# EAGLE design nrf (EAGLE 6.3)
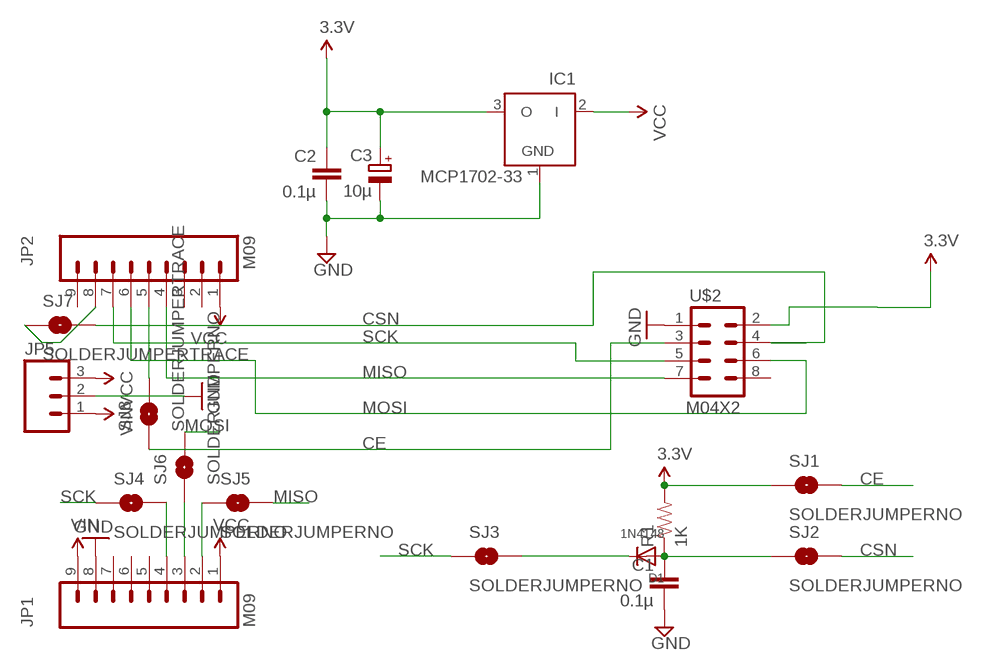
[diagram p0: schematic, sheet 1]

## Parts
C1  0.1µ  CAPPTH  [CAP-PTH-SMALL]
C2  0.1µ  CAPPTH  [CAP-PTH-SMALL]
C3  10µ  CPOL-EUE1.8-4  [E1,8-4]
D1  1N4148  DIODEDO-1N4148  [DO-1N4148]
IC1  MCP1702-33  MCP1702Z  [TO92]
JP1  M09  [1X09]
JP2  M09  [1X09]
JP5  M03PTH  [1X03]
R1  1K  RESISTORAXIAL-0.3  [AXIAL-0.3]
SJ1  SOLDERJUMPERNO  [SJ_2S-NO]
SJ2  SOLDERJUMPERNO  [SJ_2S-NO]
SJ3  SOLDERJUMPERNO  [SJ_2S-NO]
SJ4  SOLDERJUMPERNO  [SJ_2S-NO]
SJ5  SOLDERJUMPERNO  [SJ_2S-NO]
SJ6  SOLDERJUMPERNO  [SJ_2S-NO]
SJ7  SOLDERJUMPERTRACE  [SJ_2S-TRACE]
SJ8  SOLDERJUMPERTRACE  [SJ_2S-TRACE]
U$2  M04X2  [2X4]

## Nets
3.3V: C2.1 C3.+ IC1.3(O) R1.P$2 SJ1.1 U$2.2
CE: SJ1.2 SJ8.1 U$2.3
CSN: SJ2.2 SJ7.2 U$2.4
GND [POWER]: C1.2 C2.2 C3.- IC1.1(GND) JP1.8 JP5.2 U$2.1
MISO: JP2.4 SJ5.2 U$2.7
MOSI: JP2.6 SJ6.2 U$2.6
N$1: C1.1 D1.A R1.P$1 SJ2.1
N$2: JP2.8 SJ7.1
N$3: JP2.5 SJ8.2
N$7: D1.C SJ3.2
N$8: JP1.2 SJ5.1
N$9: JP1.3 SJ6.1
N$10: JP1.4 SJ4.2
SCK: JP2.7 SJ3.1 SJ4.1 U$2.5
VCC [POWER]: IC1.2(I) JP1.1 JP2.1 JP5.3
VIN [POWER]: JP1.9 JP5.1
Unconnected: JP1.5 JP1.6 JP1.7 JP2.2 JP2.3 JP2.9 U$2.8

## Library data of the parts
C1 C2 = SparkFun:CAP: Capacitor
C3 = resistor:CPOL-EU: POLARIZED CAPACITOR, European symbol
D1 = adafruit:DIODE: Diode
IC1 = JeeLabs:MCP1702: 200 mA, Low Power Low Dropout Voltage Regulator
JP1 JP2 = SparkFun:M09: Header 9 Standard 9-pin 0.1" header. Use with straight break away headers (SKU : PRT-00116), right angle break away headers (PRT-00553), swiss pins (PRT-00743), machine pins (PRT-00117), and female headers (PRT-00115).
JP5 = SparkFun:M03: Header 3 Standard 3-pin 0.1" header. Use with straight break away headers (SKU : PRT-00116), right angle break away headers (PRT-00553), swiss pins (PRT-00743), machine pins (PRT-00117), and female headers (PRT-00115). Molex polarized connector foot print use with SKU : PRT-08232 with associated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
R1 = SparkFun-Passives:RESISTOR: Resistor
SJ1-SJ8 = SparkFun-Passives:SOLDERJUMPER: Solder Jumper
U$2 = SparkFun-Connectors:M04X2: .1" header, two rows of four.

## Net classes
0 default: width 0.203 mm
1 POWER: width 0.203 mm

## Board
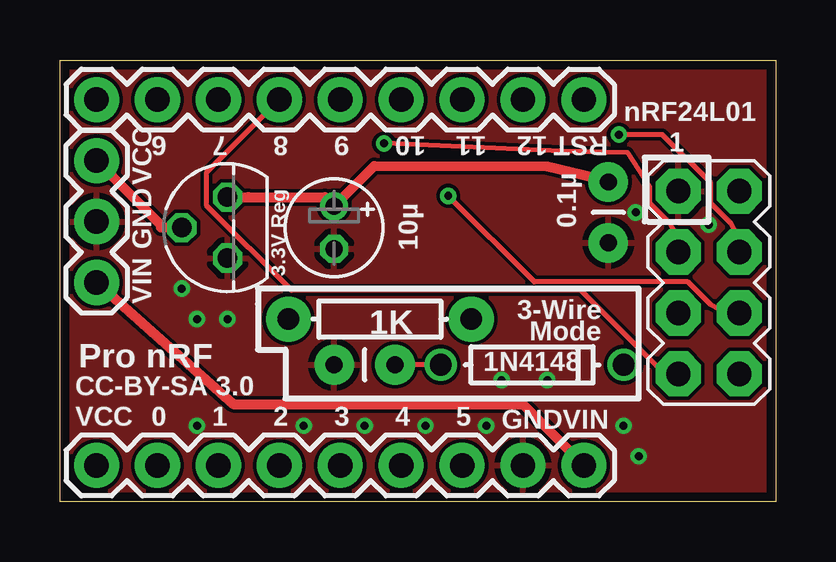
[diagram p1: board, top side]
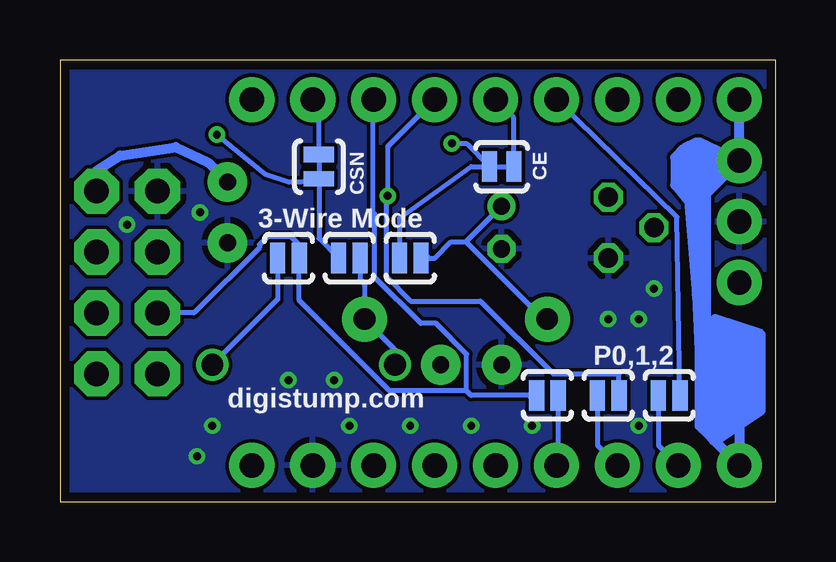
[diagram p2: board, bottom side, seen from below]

Size 29.84 x 18.41 mm. Coordinates in mm from the lower left corner, seen from the top.
Outline: 0,0 0,18.41 29.84,18.41 29.84,0 0,0
Copper layers (1*16): Top 0.0356mm / dielectric 1.5011mm / Bottom 0.0356mm
Design rules "eriks *": minimum track width 8mil, minimum drill 13mil, track to track 6mil, track to pad 6mil, pad to pad 6mil, via to via 6mil, smd to smd 6mil, copper to edge 15mil, drill to drill 6mil, minimum pad ring 7mil, minimum via ring 7mil, stop-mask expansion 4mil, vias tented up to drill 20mil, thermal gap 10mil

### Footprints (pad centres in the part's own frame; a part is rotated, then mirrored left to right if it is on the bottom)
CAP-PTH-SMALL = drill 0.7 pad 1.651: 1 0,0; 2 2.54,0
E1,8-4 = drill 0.711 pad 1.168: + -0.889,0 | drill 0.711 pad 1.168 octagon: - 0.889,0
DO-1N4148 = drill 0.9: A -3.81,0; C 3.81,0
TO92 = drill 0.813 octagon: 1 -1.27,0; 2 0,1.905; 3 1.27,0
1X09 = drill 1.016 pad 1.88: 1 0,0; 2 2.54,0; 3 5.08,0; 4 7.62,0; 5 10.16,0; 6 12.7,0; 7 15.24,0; 8 17.78,0; 9 20.32,0
1X03 = drill 1.016 pad 1.88: 1 0,0; 2 2.54,0; 3 5.08,0
AXIAL-0.3 = drill 0.9 pad 1.88: P$1 -3.81,0; P$2 3.81,0
SJ_2S-NO = smd 0.635 x 1.27: 1 -0.45,0; 2 0.45,0
SJ_2S-TRACE = smd 0.635 x 1.27: 1 -0.508,0; 2 0.508,0
2X4 = drill 1.016 pad 1.88 octagon: 1 -3.81,-1.27; 2 -3.81,1.27; 3 -1.27,-1.27; 4 -1.27,1.27; 5 1.27,-1.27; 6 1.27,1.27; 7 3.81,-1.27; 8 3.81,1.27

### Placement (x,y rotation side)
C1  13.97,5.71 180 top
C2  22.86,13.34 270 top
C3  11.43,11.43 270 top
D1  19.68,5.71 0 top
IC1  6.99,11.43 90 top
JP1  1.52,1.52 0 top
JP2  1.52,16.76 0 top
JP5  1.52,9.14 90 top
R1  13.34,7.62 180 top
SJ1  15.24,10.16 180 bottom
SJ2  17.78,10.16 180 bottom
SJ3  20.32,10.16 180 bottom
SJ4  9.53,4.45 0 bottom
SJ5  4.45,4.45 0 bottom
SJ6  6.99,4.45 0 bottom
SJ7  19.05,13.97 270 bottom
SJ8  11.43,13.97 0 bottom
U$2  27.05,9.14 270 top

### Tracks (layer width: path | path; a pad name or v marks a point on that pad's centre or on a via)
3.3V
  Top 0.203: C2.1 22.84,13.35
  Top 0.406: 22.84,13.35 20.32,13.97 13.1,13.99 C3.+ 11.05,12.7 7.85,12.7 IC1.3
  Bottom 0.203: 12.91,10.84 9.7,7.62 R1.P$2 | 12.91,10.84 13.54,10.84 14.22,10.16 14.61,10.16 SJ1.1 | C3.+ 12.91,10.84
  Bottom 0.406: U$2.2 28.32,13.79 27.34,14.43 25.01,14.78 23.67,14.15 C2.1 | SJ1.1 14.61,10.16
CE  (via drill 0.33)
  Top 0.203: U$2.3 25.78,10.97 25.44,11.61 24.59,12.46 24.59,13.13 23.67,14.56 20.95,14.61 v13.51,14.94
  Bottom 0.203: SJ1.2 15.69,11.83 12.7,13.97 SJ8.1 12.91,14.94 v13.51,14.94
  Bottom 0.406: SJ1.2
CSN  (via drill 0.33)
  Top 0.203: U$2.4 28.32,10.97 27.98,11.61 27.13,12.46 27.13,13.3 25.12,15.31 v23.3,15.31
  Bottom 0.203: SJ2.2 19.05,10.98 SJ7.2 19.81,13.34 20.32,13.34 21.27,13.65 v23.3,15.31
  Bottom 0.406: SJ2.2
GND  (via drill 0.33 pad 0.69)
  other vias: 15.24,3.17 12.7,3.17 17.78,3.17 10.16,3.17 23.5,3.17 5.71,3.17 5.71,7.62 6.99,7.62 5.08,8.89 18.41,5.08 20.32,5.08 24.13,1.91 24,12.06 27.05,11.56
  pour Top: -2.54,40.01 34.29,40.01 34.92,-5.08 -1.91,-5.08
  pour Bottom: -2.54,40.01 31.75,40.01 32.38,-2.54 -2.54,-2.54
MISO
  Top 0.203: U$2.7 25.22,5.33 24.59,5.94 21.71,8.81 9.65,8.81 6.12,12.34 6.12,13.74 JP2.4
  Bottom 0.203: SJ5.2 4.12,11.87 JP2.4
  Bottom 0.406: SJ5.2
MOSI  (via drill 0.33 pad 0.69)
  Top 0.203: v16.19,12.76 19.77,9.17 26.18,9.17 27.13,8.22 27.76,7.87 U$2.6
  Bottom 0.203: JP2.6 16.19,14.8 v16.19,12.76 16.26,12.68 16.26,9.41 15.22,8.37 12.32,8.37 9.28,5.33 6.54,5.33 SJ6.2
  Bottom 0.406: SJ6.2
N$1
  Top 0.203: D1.A C1.1
  Bottom 0.203: SJ2.1 17.33,9.27 17.14,9.09 R1.P$1 15.88,6.35 D1.A
  Bottom 0.406: SJ2.1
N$2
  Bottom 0.203: SJ7.1 19.05,16.51 JP2.8
N$3
  Bottom 0.203: SJ8.2 10.92,16 JP2.5
N$7
  Bottom 0.203: SJ3.2 20.77,8.44 D1.C
  Bottom 0.406: SJ3.2
N$8
  Bottom 0.203: SJ5.1 4.89,2.35 JP1.2
  Bottom 0.406: SJ5.1
N$9
  Bottom 0.203: SJ6.1 7.43,2.35 JP1.3
  Bottom 0.406: SJ6.1
N$10
  Bottom 0.203: SJ4.2 9.07,1.59 JP1.4
  Bottom 0.406: SJ4.2
SCK
  Bottom 0.203: 12.89,4.63 12.89,6.16 14.16,7.44 14.79,7.44 16.73,9.37 16.73,12 16.79,12.06 16.79,16.74 JP2.7 | SJ4.1 10.16,4.45 12.7,4.45 12.89,4.63 | 12.89,4.63 16.11,4.63 19.87,8.39 SJ3.1 19.87,10.71 20.21,11.05 21.2,11.05 21.53,10.72 21.53,10.6 24.25,7.87 U$2.5
  Bottom 0.406: SJ4.1 10.16,4.45 | SJ3.1
VCC
  Top 0.406: IC1.2 4.22,11.43 4.22,11.53 JP5.3
  Bottom 0.406: JP5.3 1.65,14.1 | 1.65,14.1 2.67,13.08 | 2.67,13.08 3.35,12.39 2.72,2.72 | 2.72,2.72 2.54,2.54 | 2.54,2.54 JP1.1 | JP5.3 JP2.1 | 2.54,2.54 0.64,3.81 0.64,6.99 2.54,7.62 2.54,2.54 | 2.54,2.54 0.89,3.68 0.89,3.94 | 0.89,3.94 0.89,6.86 2.29,7.24 2.16,3.05 0.89,3.94 | 0.89,3.94 1.14,6.6 2.03,6.86 1.78,3.56 1.91,3.43 1.14,4.19 1.52,6.35 1.78,6.48 1.52,4.06 JP1.1 | JP1.1 2.72,2.72 | 2.72,2.72 3.05,3.05 | 3.05,3.05 3.17,3.17 3.17,10.29 | 3.17,10.29 3.17,13.08 3.17,13.97 3.17,14.99 JP5.3 | JP5.3 2.92,14.61 2.92,14.48 | 2.92,14.48 2.92,3.3 2.92,14.48 | 2.92,14.48 1.65,14.1 | 1.65,14.1 2.67,13.08 | 2.67,13.08 2.67,14.1 2.16,13.97 2.54,13.59 3.3,14.99 3.81,14.73 4.19,14.35 4.19,13.21 3.56,12.45 3.17,10.29 | 3.17,10.29 3.3,14.73 3.94,14.22 3.94,13.21 3.43,12.83 3.56,14.35 3.68,13.34 3.3,8.64 3.05,3.05
VIN
  Top 0.406: JP5.1 7.23,4.08 19.29,4.08 JP1.9

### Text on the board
tPlace: nRF24L01 | 6 | 7 | 8 | 9 | 10 | 11 | 12 | RST | 1 | VCC | GND | 3.3V Reg | VIN | 3-Wire | Mode | Pro nRF | CC-BY-SA 3.0 | VCC | 0 | 1 | 2 | 3 | 4 | 5 | GND | VIN
bPlace: CE | CSN | 3-Wire Mode | P0,1,2 | digistump.com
